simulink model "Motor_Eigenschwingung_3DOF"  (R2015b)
settings: Solver=ode45  StartTime=0.0  StopTime=10.0  RelTol=1e-5
undefined symbols (not defined in the file): B, deg, H, kg, L, m, N, omg, s, X, XW, Y, YW, Z
libraries: sm_lib x19, nesl_utility x4

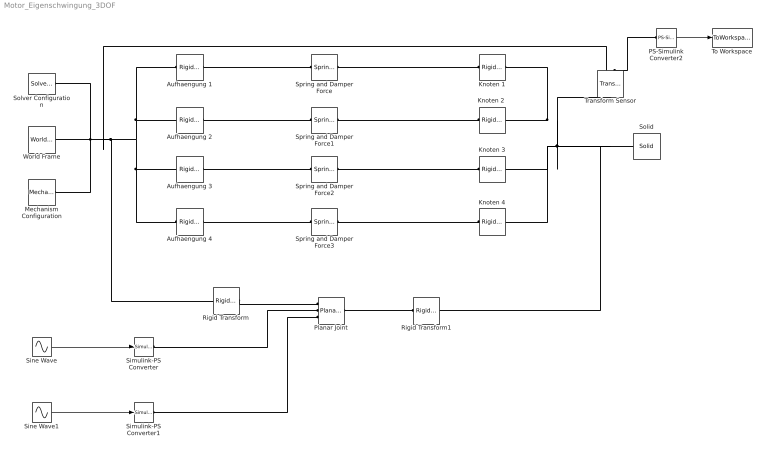
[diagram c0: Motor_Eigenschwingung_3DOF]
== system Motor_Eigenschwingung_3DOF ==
  Aufhaengung 1 : sm_lib/Frames and Transforms/Rigid Transform  TranslationMethod=Cartesian  TranslationLengthUnit=mm  TranslationStandardAxis=+X  TranslationStandardOffset=L/2  TranslationCartesianOffset=[XW YW 0]  TranslationROffset=0  TranslationROffsetUnits=m  TranslationZOffset=0  TranslationZOffsetUnits=m  TranslationThetaOffset=0  TranslationThetaOffsetUnits=deg  RotationMethod=None  RotationAngleUnits=deg  RotationStandardAxis=+Z  RotationAngle=0.0  RotationArbitraryAxis=[0 0 1]  FollAlignAxisA=+X  BaseAlignAxisA=+Y  FollAlignAxisB=+Y  BaseAlignAxisB=+Z  RotationSequenceAxes=FollowerAxes  RotationSequence=XYX  RotationSequenceAngles=[0 0 0]  RotationSequenceAnglesUnits=deg  RotationMatrix=[1 0 0; 0 1 0; 0 0 1]  BlockFunction=simmechanics.library.frames_transforms.rigid_transform
  Aufhaengung 2 : sm_lib/Frames and Transforms/Rigid Transform  TranslationMethod=Cartesian  TranslationLengthUnit=mm  TranslationStandardAxis=+Y  TranslationStandardOffset=B/2  TranslationCartesianOffset=[XW -YW 0]  TranslationROffset=0  TranslationROffsetUnits=m  TranslationZOffset=0  TranslationZOffsetUnits=m  TranslationThetaOffset=0  TranslationThetaOffsetUnits=deg  RotationMethod=None  RotationAngleUnits=deg  RotationStandardAxis=+Z  RotationAngle=0.0  RotationArbitraryAxis=[0 0 1]  FollAlignAxisA=+X  BaseAlignAxisA=+Y  FollAlignAxisB=+Y  BaseAlignAxisB=+Z  RotationSequenceAxes=FollowerAxes  RotationSequence=XYX  RotationSequenceAngles=[0 0 0]  RotationSequenceAnglesUnits=deg  RotationMatrix=[1 0 0; 0 1 0; 0 0 1]  BlockFunction=simmechanics.library.frames_transforms.rigid_transform
  Aufhaengung 3 : sm_lib/Frames and Transforms/Rigid Transform  TranslationMethod=Cartesian  TranslationLengthUnit=mm  TranslationStandardAxis=-X  TranslationStandardOffset=B/2  TranslationCartesianOffset=[-XW -YW 0]  TranslationROffset=0  TranslationROffsetUnits=m  TranslationZOffset=0  TranslationZOffsetUnits=m  TranslationThetaOffset=0  TranslationThetaOffsetUnits=deg  RotationMethod=None  RotationAngleUnits=deg  RotationStandardAxis=+Z  RotationAngle=0.0  RotationArbitraryAxis=[0 0 1]  FollAlignAxisA=+X  BaseAlignAxisA=+Y  FollAlignAxisB=+Y  BaseAlignAxisB=+Z  RotationSequenceAxes=FollowerAxes  RotationSequence=XYX  RotationSequenceAngles=[0 0 0]  RotationSequenceAnglesUnits=deg  RotationMatrix=[1 0 0; 0 1 0; 0 0 1]  BlockFunction=simmechanics.library.frames_transforms.rigid_transform
  Aufhaengung 4 : sm_lib/Frames and Transforms/Rigid Transform  TranslationMethod=Cartesian  TranslationLengthUnit=mm  TranslationStandardAxis=-Y  TranslationStandardOffset=B/2  TranslationCartesianOffset=[-XW YW 0]  TranslationROffset=0  TranslationROffsetUnits=m  TranslationZOffset=0  TranslationZOffsetUnits=m  TranslationThetaOffset=0  TranslationThetaOffsetUnits=deg  RotationMethod=None  RotationAngleUnits=deg  RotationStandardAxis=+Z  RotationAngle=0.0  RotationArbitraryAxis=[0 0 1]  FollAlignAxisA=+X  BaseAlignAxisA=+Y  FollAlignAxisB=+Y  BaseAlignAxisB=+Z  RotationSequenceAxes=FollowerAxes  RotationSequence=XYX  RotationSequenceAngles=[0 0 0]  RotationSequenceAnglesUnits=deg  RotationMatrix=[1 0 0; 0 1 0; 0 0 1]  BlockFunction=simmechanics.library.frames_transforms.rigid_transform
  Knoten 1 : sm_lib/Frames and Transforms/Rigid Transform  TranslationMethod=Cartesian  TranslationLengthUnit=mm  TranslationStandardAxis=+X  TranslationStandardOffset=L/2  TranslationCartesianOffset=[L/2 B/2 0]  TranslationROffset=0  TranslationROffsetUnits=m  TranslationZOffset=0  TranslationZOffsetUnits=m  TranslationThetaOffset=0  TranslationThetaOffsetUnits=deg  RotationMethod=None  RotationAngleUnits=deg  RotationStandardAxis=+Z  RotationAngle=0.0  RotationArbitraryAxis=[0 0 1]  FollAlignAxisA=+X  BaseAlignAxisA=+Y  FollAlignAxisB=+Y  BaseAlignAxisB=+Z  RotationSequenceAxes=FollowerAxes  RotationSequence=XYX  RotationSequenceAngles=[0 0 0]  RotationSequenceAnglesUnits=deg  RotationMatrix=[1 0 0; 0 1 0; 0 0 1]  BlockFunction=simmechanics.library.frames_transforms.rigid_transform
  "Knoten 2 " : sm_lib/Frames and Transforms/Rigid Transform  TranslationMethod=Cartesian  TranslationLengthUnit=mm  TranslationStandardAxis=+Y  TranslationStandardOffset=B/2  TranslationCartesianOffset=[L/2 -B/2 0]  TranslationROffset=0  TranslationROffsetUnits=m  TranslationZOffset=0  TranslationZOffsetUnits=m  TranslationThetaOffset=0  TranslationThetaOffsetUnits=deg  RotationMethod=None  RotationAngleUnits=deg  RotationStandardAxis=+Z  RotationAngle=0.0  RotationArbitraryAxis=[0 0 1]  FollAlignAxisA=+X  BaseAlignAxisA=+Y  FollAlignAxisB=+Y  BaseAlignAxisB=+Z  RotationSequenceAxes=FollowerAxes  RotationSequence=XYX  RotationSequenceAngles=[0 0 0]  RotationSequenceAnglesUnits=deg  RotationMatrix=[1 0 0; 0 1 0; 0 0 1]  BlockFunction=simmechanics.library.frames_transforms.rigid_transform
  Knoten 3 : sm_lib/Frames and Transforms/Rigid Transform  TranslationMethod=Cartesian  TranslationLengthUnit=mm  TranslationStandardAxis=-X  TranslationStandardOffset=B/2  TranslationCartesianOffset=[-L/2 -B/2 0]  TranslationROffset=0  TranslationROffsetUnits=m  TranslationZOffset=0  TranslationZOffsetUnits=m  TranslationThetaOffset=0  TranslationThetaOffsetUnits=deg  RotationMethod=None  RotationAngleUnits=deg  RotationStandardAxis=+Z  RotationAngle=0.0  RotationArbitraryAxis=[0 0 1]  FollAlignAxisA=+X  BaseAlignAxisA=+Y  FollAlignAxisB=+Y  BaseAlignAxisB=+Z  RotationSequenceAxes=FollowerAxes  RotationSequence=XYX  RotationSequenceAngles=[0 0 0]  RotationSequenceAnglesUnits=deg  RotationMatrix=[1 0 0; 0 1 0; 0 0 1]  BlockFunction=simmechanics.library.frames_transforms.rigid_transform
  Knoten 4 : sm_lib/Frames and Transforms/Rigid Transform  TranslationMethod=Cartesian  TranslationLengthUnit=mm  TranslationStandardAxis=-Y  TranslationStandardOffset=B/2  TranslationCartesianOffset=[-L/2 B/2 0]  TranslationROffset=0  TranslationROffsetUnits=m  TranslationZOffset=0  TranslationZOffsetUnits=m  TranslationThetaOffset=0  TranslationThetaOffsetUnits=deg  RotationMethod=None  RotationAngleUnits=deg  RotationStandardAxis=+Z  RotationAngle=0.0  RotationArbitraryAxis=[0 0 1]  FollAlignAxisA=+X  BaseAlignAxisA=+Y  FollAlignAxisB=+Y  BaseAlignAxisB=+Z  RotationSequenceAxes=FollowerAxes  RotationSequence=XYX  RotationSequenceAngles=[0 0 0]  RotationSequenceAnglesUnits=deg  RotationMatrix=[1 0 0; 0 1 0; 0 0 1]  BlockFunction=simmechanics.library.frames_transforms.rigid_transform
  Mechanism Configuration : sm_lib/Utilities/Mechanism Configuration  UniformGravity=Constant  GravityVector=[0 0 -9.80665]  GravityUnits=m/s^2  LinearizationDelta=0.001  BlockFunction=simmechanics.library.utilities.mechanism_configuration
  PS-Simulink Converter2 : nesl_utility/PS-Simulink Converter  PhysicalDomain=network_engine_domain  SubClassName=ps_output  LeftPortType=input  RightPortType=output  PseudoPeriodic=off  Frequencies=[]  Unit=1  AffineConversion=off
  Planar Joint : sm_lib/Joints/Planar Joint  SenseConstraintForce=off  SenseConstraintForceX=off  SenseConstraintForceY=off  SenseConstraintForceZ=off  SenseConstraintTorque=off  SenseConstraintTorqueX=off  SenseConstraintTorqueY=off  SenseConstraintTorqueZ=off  SenseTotalForce=off  SenseTotalForceX=off  SenseTotalForceY=off  SenseTotalForceZ=off  SenseTotalTorque=off  SenseTotalTorqueX=off  SenseTotalTorqueY=off  SenseTotalTorqueZ=off  CompositeWrenchDir=FollowerOnBase  CompositeWrenchFrame=BaseFrame  PxEquilibriumPosition=0  PxEquilibriumPositionUnits=m  PxSpringStiffness=0  PxSpringStiffnessUnits=N/m  PxDampingCoefficient=0  PxDampingCoefficientUnits=N/(m/s)  PxTorqueActuationMode=InputTorque  PxMotionActuationMode=ComputedMotion  PxSensePosition=off  PxSenseVelocity=off  PxSenseAcceleration=off  PxSenseTorqueForce=off  PxPositionTargetSpecify=on  PxPositionTargetPriority=High  PxPositionTargetValue=z_ver  PxPositionTargetValueUnits=mm  PxVelocityTargetSpecify=off  PxVelocityTargetPriority=High  PxVelocityTargetValue=0  PxVelocityTargetValueUnits=m/s  PyEquilibriumPosition=0  PyEquilibriumPositionUnits=m  PySpringStiffness=0  PySpringStiffnessUnits=N/m  PyDampingCoefficient=0  PyDampingCoefficientUnits=N/(m/s)  PyTorqueActuationMode=InputTorque  PyMotionActuationMode=ComputedMotion  PySensePosition=off  PySenseVelocity=off  PySenseAcceleration=off  PySenseTorqueForce=off  PyPositionTargetSpecify=on  PyPositionTargetPriority=High  PyPositionTargetValue=y_ver  PyPositionTargetValueUnits=mm  PyVelocityTargetSpecify=off  PyVelocityTargetPriority=High  PyVelocityTargetValue=0  PyVelocityTargetValueUnits=m/s  RzEquilibriumPosition=0  RzEquilibriumPositionUnits=deg  RzSpringStiffness=0  RzSpringStiffnessUnits=N*m/deg  RzDampingCoefficient=0  RzDampingCoefficientUnits=N*m/(deg/s)  RzTorqueActuationMode=NoTorque  RzMotionActuationMode=ComputedMotion  RzSensePosition=off  RzSenseVelocity=off  RzSenseAcceleration=off  RzSenseTorqueForce=off  RzPositionTargetSpecify=off  RzPositionTargetPriority=High  RzPositionTargetValue=0  RzPositionTargetValueUnits=deg  RzVelocityTargetSpecify=off  RzVelocityTargetPriority=High  RzVelocityTargetValue=0  RzVelocityTargetValueUnits=deg/s  BlockFunction=simmechanics.library.joints.planar_joint
  Rigid Transform : sm_lib/Frames and Transforms/Rigid Transform  TranslationMethod=None  TranslationLengthUnit=m  TranslationStandardAxis=+Z  TranslationStandardOffset=0  TranslationCartesianOffset=[0 0 0]  TranslationROffset=0  TranslationROffsetUnits=m  TranslationZOffset=0  TranslationZOffsetUnits=m  TranslationThetaOffset=0  TranslationThetaOffsetUnits=deg  RotationMethod=StandardAxis  RotationAngleUnits=deg  RotationStandardAxis=+Y  RotationAngle=90  RotationArbitraryAxis=[0 0 1]  FollAlignAxisA=+X  BaseAlignAxisA=+Y  FollAlignAxisB=+Y  BaseAlignAxisB=+Z  RotationSequenceAxes=FollowerAxes  RotationSequence=XYX  RotationSequenceAngles=[0 0 0]  RotationSequenceAnglesUnits=deg  RotationMatrix=[1 0 0; 0 1 0; 0 0 1]  BlockFunction=simmechanics.library.frames_transforms.rigid_transform
  Rigid Transform1 : sm_lib/Frames and Transforms/Rigid Transform  TranslationMethod=None  TranslationLengthUnit=m  TranslationStandardAxis=+Z  TranslationStandardOffset=0  TranslationCartesianOffset=[0 0 0]  TranslationROffset=0  TranslationROffsetUnits=m  TranslationZOffset=0  TranslationZOffsetUnits=m  TranslationThetaOffset=0  TranslationThetaOffsetUnits=deg  RotationMethod=StandardAxis  RotationAngleUnits=deg  RotationStandardAxis=+Y  RotationAngle=-90  RotationArbitraryAxis=[0 0 1]  FollAlignAxisA=+X  BaseAlignAxisA=+Y  FollAlignAxisB=+Y  BaseAlignAxisB=+Z  RotationSequenceAxes=FollowerAxes  RotationSequence=XYX  RotationSequenceAngles=[0 0 0]  RotationSequenceAnglesUnits=deg  RotationMatrix=[1 0 0; 0 1 0; 0 0 1]  BlockFunction=simmechanics.library.frames_transforms.rigid_transform
  Simulink-PS Converter : nesl_utility/Simulink-PS Converter  PhysicalDomain=network_engine_domain  SubClassName=ps_input  LeftPortType=input  RightPortType=output  PseudoPeriodic=off  Frequencies=[]  NoiseDistribution=none  NoiseParameters=[]  Unit=N  AffineConversion=off  InputFiltering=off  SimscapeFilterOrder=1  InputFilterTimeConstant=0.001  UdotUserProvided=1
  Simulink-PS Converter1 : nesl_utility/Simulink-PS Converter  PhysicalDomain=network_engine_domain  SubClassName=ps_input  LeftPortType=input  RightPortType=output  PseudoPeriodic=off  Frequencies=[]  NoiseDistribution=none  NoiseParameters=[]  Unit=N  AffineConversion=off  InputFiltering=off  SimscapeFilterOrder=1  InputFilterTimeConstant=0.001  UdotUserProvided=1
  Sine Wave : Sin  Frequency=omg  SampleTime=0
  Sine Wave1 : Sin  Frequency=omg  Phase=-pi/2  SampleTime=0
  Solid : sm_lib/Body Elements/Solid  InertiaType=CalculateFromGeometry  Mass=m  MassUnits=kg  CenterOfMass=[0 0 0]  CenterOfMassUnits=m  MomentsOfInertia=[1 1 1]  MomentsOfInertiaUnits=kg*m^2  ProductsOfInertia=[0 0 0]  ProductsOfInertiaUnits=kg*m^2  DensityBased=off  Density=1000  DensityUnits=kg/(m^3)  DoExposeReferenceFrame=on  SerializedFrames=<Frames/>  GraphicType=FromGeometry  MarkerShape=Sphere  MarkerSize=10  GraphicVisPropType=SimpleVisualProperties  GraphicDiffuseColor=RGB_Block  GraphicSpecularColor=[0.5 0.5 0.5 1.0]  GraphicAmbientColor=[0.15 0.15 0.15 1.0]  GraphicEmissiveColor=[0.0 0.0 0.0 1.0]  GraphicShininess=75  GraphicOpacity=1.0  GeometryShape=Brick  RectangleSize=[1 1]  RectangleSizeUnits=m  BrickDimensions=[L B H]  BrickDimensionUnits=mm  CylinderRadius=1  CylinderRadiusUnits=m  CylinderLength=1  CylinderLengthUnits=m  SphereRadius=1  SphereRadiusUnits=m  EllipsoidRadii=[1 1 1]  EllipsoidRadiiUnits=m  ExtrusionCrossSection=[1 1; -1 1; -1 -1; 1 -1]  ExtrusionCrossSectionUnits=m  ExtrusionLength=1  ExtrusionLengthUnits=m  PolygonNumSides=3  PolygonOuterRadius=1  PolygonOuterRadiusUnits=m  ExtGeomFileType=STL  ExtGeomFileUnits=m  RevolutionCrossSection=[1 1; 1 -1; 2 -1; 2 1]  RevolutionCrossSectionUnits=m  RevolutionExtent=Full  RevolutionAngle=180  RevolutionAngleUnits=deg  BlockFunction=simmechanics.library.body_elements.solid
  Solver Configuration : nesl_utility/Solver Configuration  PhysicalDomain=network_engine_domain  SubClassName=solver  LeftPortType=input  RightPortType=generic  Accelerate=off  Tones=[]  Harmonics=[]  SimulateNoise=off  Profile=off  UseLocalSampling=off  EnableSwitchedLinearOptims=on  FrequencyDomain=off  UseCCode=off  RelTol=0.001  AbsTol=1e-06  MinStep=1e-09  ToWorkspace=off  RevertToSquareIcSolve=off  NumHomotopyIterations=100  PhasorMode=off  PhasorModeNumHarmonics=1  DoDC=off  ResidualTolerance=1e-09  UseLocalSolver=off  LocalSolverChoice=NE_BACKWARD_EULER_ADVANCER  LocalSolverSampleTime=0.001  DoFixedCost=off  MaxNonlinIter=3  MaxModeIter=2  LinearAlgebra=Sparse  DelaysMemoryBudget=1024  AutomaticFiltering=on  FilteringTimeConstant=0.001
  Spring and Damper Force{,1..3} (4 alike) : sm_lib/Forces and Torques/Spring and Damper Force  NaturalLength=L0  NaturalLengthUnits=mm  SpringStiffness=c  SpringStiffnessUnits=N/m  DampingCoefficient=b  DampingCoefficientUnits=N/(m/s)  SenseForce=off  BlockFunction=simmechanics.library.forces_torques.spring_damper_force
  To Workspace : ToWorkspace  VariableName=Weg  SaveFormat=Timeseries  SampleTime=-1
  Transform Sensor : sm_lib/Frames and Transforms/Transform Sensor  MeasurementFrame=World  SenseAngle=off  SenseAxis=off  SenseAngle1=off  SenseAngle2=off  SenseAngle3=off  SenseQ=off  SenseR=off  SenseOmegaX=off  SenseOmegaY=off  SenseOmegaZ=off  SenseOmega1=off  SenseOmega2=off  SenseOmega3=off  SenseQDot=off  SenseRDot=off  SenseAlphaX=off  SenseAlphaY=off  SenseAlphaZ=off  SenseAlpha1=off  SenseAlpha2=off  SenseAlpha3=off  SenseQDDot=off  SenseRDDot=off  SenseX=off  SenseY=off  SenseZ=on  SenseRad=off  SenseAzim=off  SenseDist=off  SenseInc=off  SenseXDot=off  SenseYDot=off  SenseZDot=off  SenseRadDot=off  SenseAzimDot=off  SenseDistDot=off  SenseIncDot=off  SenseXDDot=off  SenseYDDot=off  SenseZDDot=off  SenseRadDDot=off  SenseAzimDDot=off  SenseDistDDot=off  SenseIncDDot=off  BlockFunction=simmechanics.library.frames_transforms.transform_sensor
  World Frame : sm_lib/Frames and Transforms/World Frame  BlockFunction=simmechanics.library.frames_transforms.world_frame
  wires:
  PS-Simulink Converter2/1 -> To Workspace/1
  Sine Wave/1 -> Simulink-PS Converter/1
  Sine Wave1/1 -> Simulink-PS Converter1/1
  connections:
  Knoten 1/LConn1 -- Rigid Transform1/RConn1 -- Solid/RConn1 -- Transform Sensor/LConn1 -- Knoten 4/LConn1 -- Knoten 3/LConn1 -- "Knoten 2 "/LConn1
  Aufhaengung 1/RConn1 -- Spring and Damper Force/LConn1
  Spring and Damper Force/RConn1 -- Knoten 1/RConn1
  Aufhaengung 2/RConn1 -- Spring and Damper Force1/LConn1
  Spring and Damper Force1/RConn1 -- "Knoten 2 "/RConn1
  Spring and Damper Force2/RConn1 -- Knoten 3/RConn1
  Spring and Damper Force3/RConn1 -- Knoten 4/RConn1
  Spring and Damper Force3/LConn1 -- Aufhaengung 4/RConn1
  Spring and Damper Force2/LConn1 -- Aufhaengung 3/RConn1
  PS-Simulink Converter2/LConn1 -- Transform Sensor/RConn2
  Aufhaengung 1/LConn1 -- Aufhaengung 2/LConn1 -- Aufhaengung 3/LConn1 -- Aufhaengung 4/LConn1 -- Rigid Transform/LConn1 -- Transform Sensor/RConn1 -- Mechanism Configuration/RConn1 -- World Frame/RConn1 -- Solver Configuration/RConn1
  Rigid Transform/RConn1 -- Planar Joint/LConn1
  Planar Joint/RConn1 -- Rigid Transform1/LConn1
  Simulink-PS Converter/RConn1 -- Planar Joint/LConn2
  Simulink-PS Converter1/RConn1 -- Planar Joint/LConn3
